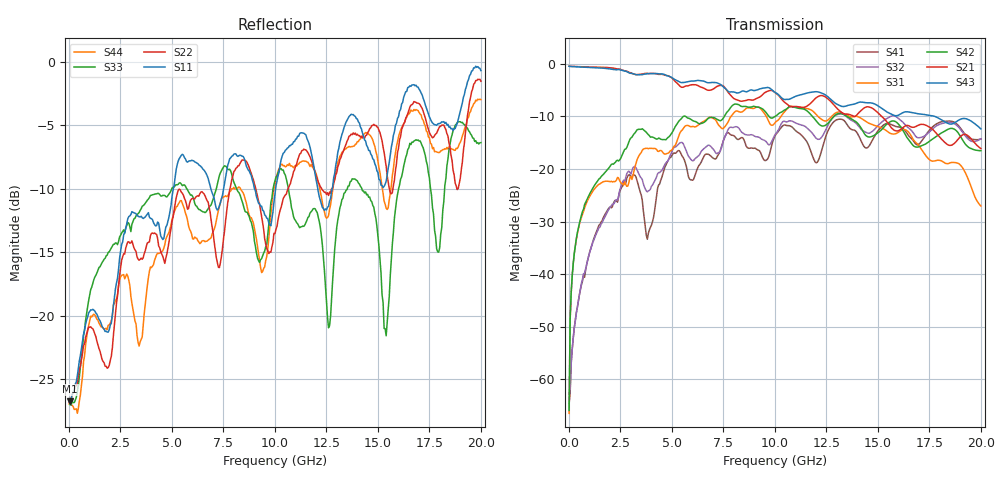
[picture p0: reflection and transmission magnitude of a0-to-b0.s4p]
!Agilent Technologies,N5225A,MY51451112,A.09.50.13
!Agilent N5225A: A.09.50.13
!Date: Wednesday, May 23, 2018 06:37:58
!Correction: S11(Full 4 Port(1,2,3,4))
!S12(Full 4 Port(1,2,3,4))
!S13(Full 4 Port(1,2,3,4))
!S14(Full 4 Port(1,2,3,4))
!S21(Full 4 Port(1,2,3,4))
!S22(Full 4 Port(1,2,3,4))
!S23(Full 4 Port(1,2,3,4))
!S24(Full 4 Port(1,2,3,4))
!S31(Full 4 Port(1,2,3,4))
!S32(Full 4 Port(1,2,3,4))
!S33(Full 4 Port(1,2,3,4))
!S34(Full 4 Port(1,2,3,4))
!S41(Full 4 Port(1,2,3,4))
!S42(Full 4 Port(1,2,3,4))
!S43(Full 4 Port(1,2,3,4))
!S44(Full 4 Port(1,2,3,4))
!S4P File: Measurements: <S11,S12,S13,S14>,
!<S21,S22,S23,S24>,
!<S31,S32,S33,S34>,
!<S41,S42,S43,S44>:
# Hz S  RI  R 50
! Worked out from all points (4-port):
!   401 points, 10 MHz to 20 GHz, reference 50 ohm
!   strongest paths, dB at 10 MHz, 5.008 GHz, 10.01 GHz, 15 GHz, 20 GHz:
!     S43: -0.5, -2.6, -5.4, -8.0, -12.4
!     S21: -0.4, -2.7, -5.5, -9.3, -16.1
!     S42: -65.9, -13.1, -10.0, -13.1, -16.5
!     S31: -66.5, -16.3, -11.2, -11.9, -27.0
!     S32: -62.8, -16.6, -13.5, -11.7, -14.3
!     S41: -64.6, -17.4, -13.7, -12.7, -14.3
!   lowest |S11| = -26.7 dB at 59.98 MHz (marker M1), VSWR 1.10, Z = 54.8 - j0.64 ohm
!   |S11| at or under -10 dB: start of sweep to 5.071 GHz; 9.006 GHz to 10.04 GHz (1.031 GHz wide, 10.8 % of centre); 12.08 GHz to 12.78 GHz (703 MHz wide, 5.65 % of centre)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
1e7  0.0453 -0.00986  0.9475 0.00247  0.000499 0.000187  0.000527 -0.00109
     0.9511 0.00338  0.0446 -0.0102  0.000172 -0.000449  0.00027 0.000181
     0.000275 0.000388  0.000461 -0.000555  0.045 -0.0106  0.949 0.00234
     0.000239 -0.000535  0.000238 0.000446  0.9491 0.00198  0.0438 -0.01
5.9975e7  0.0456 -0.00583  0.9457 -0.0292  0.000558 0.00362  0.000294 -0.000769
          0.9483 -0.0291  0.0457 -0.00576  0.00019 -0.000603  0.000573 0.00365
          0.00055 0.00366  0.000217 -0.000774  0.0441 -0.00612  0.9453 -0.0317
          0.000262 -0.000699  0.000414 0.00376  0.9455 -0.0322  0.0449 -0.00441
6.59675e8  0.0187 -0.0773  0.9057 -0.2317  0.0121 0.0352  -0.00118 -0.00849
           0.9084 -0.232  0.0125 -0.0698  -0.000516 -0.00908  0.00618 0.0391
           0.0121 0.0352  -0.000547 -0.00896  0.0166 -0.073  0.8977 -0.2428
           -0.00122 -0.00851  0.00617 0.039  0.8979 -0.2431  0.0032 -0.0574
3.358325e9  -0.2442 -0.0332  0.4108 -0.6747  0.0517 0.1181  -0.0388 0.0601
            0.4116 -0.6777  -0.1554 -0.0611  -0.0866 0.0353  0.1181 0.2073
            0.052 0.1182  -0.0864 0.0353  -0.2331 -0.0962  0.3854 -0.6873
            -0.0388 0.0603  0.1181 0.2069  0.3853 -0.6876  -0.0784 -0.00334
1.2004e10  0.252 0.2299  -0.4373 -0.1841  0.2295 -0.2363  0.1138 0.0127
           -0.4397 -0.1828  0.201 0.2914  0.1961 0.0137  0.2351 -0.1648
           0.2289 -0.2379  0.1959 0.0135  -0.0859 0.2435  -0.5426 -0.035
           0.114 0.012  0.2345 -0.1654  -0.5429 -0.0337  0.1812 0.3118
1.54023e10  0.2847 -0.1827  -0.1841 0.2177  0.0224 -0.231  0.2009 -0.1797
            -0.1837 0.2195  0.3542 0.1554  0.2308 -0.1917  0.115 -0.2379
            0.0212 -0.2316  0.2303 -0.192  0.0784 -0.0282  -0.2041 0.2872
            0.2 -0.1817  0.1139 -0.2383  -0.2035 0.2879  0.2646 0.0097
2e10  0.5807 -0.716  0.0947 0.1238  -0.0177 -0.0408  -0.0999 -0.1648
      0.0962 0.1234  0.5832 -0.5998  -0.0984 -0.167  -0.1306 -0.0723
      -0.0182 -0.0407  -0.0984 -0.1668  0.1133 -0.4661  0.192 0.1445
      -0.1021 -0.164  -0.1309 -0.0717  0.1927 0.144  0.5079 -0.4938
